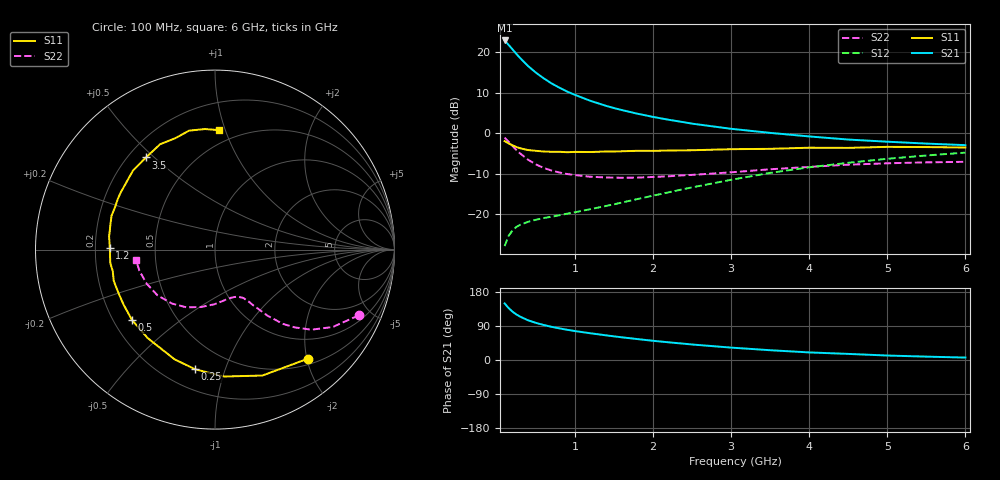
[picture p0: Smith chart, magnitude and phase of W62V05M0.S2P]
! SIEMENS Small Signal Semiconductors
! BFR193W
! Si NPN RF Bipolar Junction Transistor in SOT323
! VCE = 2 V  IC = 5 mA
! Common Emitter S-Parameters:  September  1992
# GHz  S  MA  R  50
!  f  S11  S21  S12  S22
! GHz  MAG  ANG  MAG  ANG  MAG  ANG  MAG  ANG
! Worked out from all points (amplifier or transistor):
!   28 points, 100 MHz to 6 GHz, reference 50 ohm
!   highest |S21| = 22.8 dB at 100 MHz (marker M1)
!   |S21| within 3 dB of that: start of sweep to 237 MHz
!   unconditionally stable (mu >= 1): 1.174 GHz to 2.585 GHz
!   at 300 MHz: K = 0.36, MSG = 20.5 dB, |S12| = -22.5 dB
!   at 1.5 GHz: K = 1.07, MAG = 10.2 dB, |S12| = -17.5 dB
!   at 6 GHz: K = 0.92, MSG = 0.9 dB, |S12| = -4.8 dB
!   lowest NFmin = 1.20 dB at 450 MHz
!   S11 on the Smith chart (normalised r, x): 100 MHz: 0.60, -2.03; 250 MHz: 0.32, -0.79; 500 MHz: 0.28, -0.34; 1.2 GHz: 0.26, +0.01; 3.5 GHz: 0.27, +0.47; 6 GHz: 0.40, +0.95
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0.1  0.7992 -49.4  13.81 149.3  0.0407 65.5  0.8803 -24.6
0.15  0.7497 -69.4  12.22 137.3  0.0541 57.1  0.7853 -33.3
0.2  0.7089 -85.9  10.77 127.7  0.0635 50.9  0.6983 -39.7
0.25  0.6759 -99.4  9.457 120.3  0.0701 46.7  0.6206 -44.3
0.3  0.6516 -110.2  8.366 114.3  0.0746 44.0  0.5618 -47.5
0.4  0.6194 -127.3  6.701 104.8  0.0811 40.9  0.4713 -51.5
0.5  0.6064 -139.7  5.555 98.0  0.0859 40.1  0.4132 -53.7
0.6  0.5945 -149.1  4.73 92.4  0.0903 40.4  0.3731 -55.7
0.7  0.5895 -156.4  4.096 87.6  0.0937 41.4  0.3471 -56.9
0.8  0.5904 -162.9  3.631 83.5  0.0976 42.9  0.3283 -58.4
0.9  0.5823 -168.1  3.251 79.8  0.1022 44.6  0.3143 -59.4
1  0.5882 -172.7  2.958 76.4  0.1063 46.3  0.305 -61.0
1.2  0.586 179.2  2.495 70.5  0.1162 49.6  0.2908 -64.5
1.4  0.5948 172.8  2.166 65.0  0.1273 52.8  0.2849 -68.2
1.6  0.5984 167.3  1.925 59.9  0.14 55.5  0.2825 -72.2
1.8  0.6066 162.0  1.735 55.2  0.1545 57.7  0.2839 -76.7
2.2  0.611 152.2  1.461 46.7  0.187 60.7  0.2948 -85.3
3  0.6348 136.0  1.131 32.7  0.2666 61.2  0.3297 -103.9
3.5  0.6413 126.8  1.008 25.8  0.3246 58.6  0.3595 -116.6
4.5  0.6588 109.6  0.834 16.1  0.4321 49.9  0.4094 -141.5
5.5  0.674 94.7  0.744 8.9  0.5314 39.8  0.4373 -164.3
6  0.6657 88.1  0.712 6.4  0.5759 34.1  0.444 -172.7
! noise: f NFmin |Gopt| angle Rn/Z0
0.45  1.2  0.26  102  0.14
0.9  1.25  0.38  145  0.12
1.8  2.05  0.56  -161  0.12
